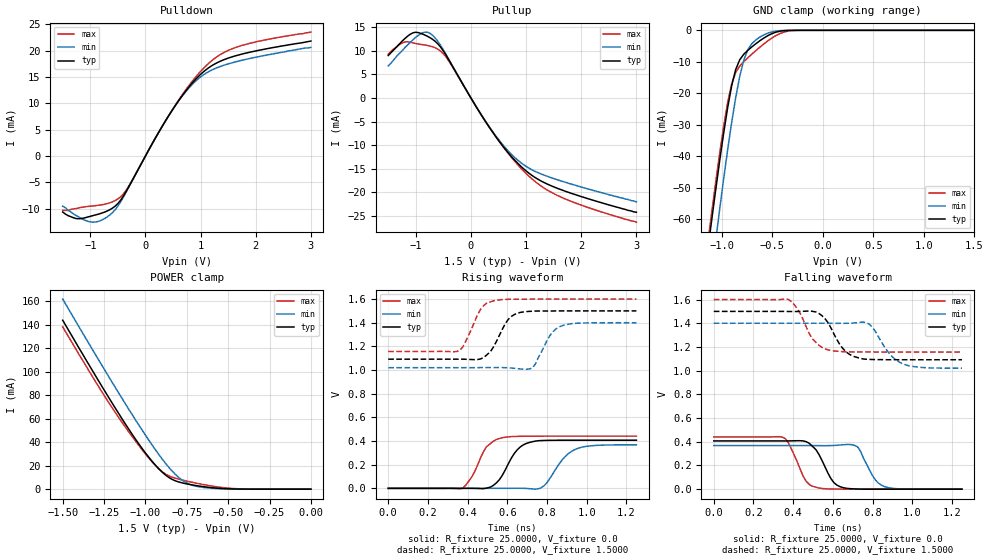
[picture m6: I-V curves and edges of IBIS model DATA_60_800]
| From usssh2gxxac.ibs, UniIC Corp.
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|   Model DATA_60_800
[Model]  DATA_60_800
Model_type I/O
Polarity   Non-Inverting
Enable   Active-High
Vinl =   0.60000000V
Vinh =   0.90000000V
Vmeas =   0.750000000V
Rref =   25.00000000
Vref =   0.75000000V
C_comp   1.6160pF   1.5990pF   1.6430pF
[Temperature Range]   25.0000   95.0000   0.0
[Voltage Range]   1.5000V   1.4000V   1.6000V
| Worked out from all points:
|   slope of the pulldown table from 0 to 0.225 V, typ, clamps not added: 53.4 ohm
|   slope of the pullup table from 0 to 0.225 V, typ, clamps not added: 52.6 ohm
|   GND clamp passes 1 mA (typ) near -0.50 V on its own axis
|   POWER clamp passes 1 mA (typ) near -0.58 V on its own axis
|   rising waveform, R_fixture 25.0000, V_fixture 0.0: 20-80 % time 86.5ps typ, 98.3ps min, 79.3ps max; typ from 0 V to 0.407 V
|   rising waveform, R_fixture 25.0000, V_fixture 1.5000: 20-80 % time 78.8ps typ, 76.2ps min, 73.4ps max; typ from 1.09 V to 1.5 V
|   falling waveform, R_fixture 25.0000, V_fixture 0.0: 20-80 % time 75.8ps typ, 70.4ps min, 70.8ps max; typ from 0.407 V to 0 V
|   falling waveform, R_fixture 25.0000, V_fixture 1.5000: 20-80 % time 88.4ps typ, 97.1ps min, 85.7ps max; typ from 1.5 V to 1.09 V
[Pulldown]
|Voltage   I(typ)   I(min)   I(max)
-1.5V     -10.6mA    -9.5mA     -10.3mA
-1.25V    -11.86mA   -11.3mA    -9.93mA
-1V       -11.42mA   -12.48mA   -9.5mA
-800mV    -10.84mA   -12.17mA   -9.25mA
-600mV    -9.882mA   -10.74mA   -8.682mA
-350mV    -6.704mA   -6.838mA   -6.505mA
200mV     3.763mA    3.796mA    3.76mA
550mV     9.696mA    9.684mA    9.781mA
850mV     13.86mA    13.59mA    14.19mA
1.15V     16.76mA    16.02mA    17.61mA
1.75V     19.33mA    18.16mA    20.97mA
3V        21.8mA     20.6mA     23.5mA
[Pullup]
|Voltage   I(typ)   I(min)   I(max)
-1.5V     9mA        6.8mA      9.3mA
-1.25V    12.03mA    10mA       11.63mA
-1.05V    13.82mA    12.36mA    11.68mA
-900mV    13.65mA    13.69mA    11.34mA
-750mV    12.84mA    13.77mA    11.04mA
-600mV    11.47mA    12.01mA    10.35mA
-450mV    9.041mA    9.198mA    8.665mA
300mV     -5.62mA    -5.548mA   -5.6mA
850mV     -13.84mA   -13.18mA   -14.16mA
1.2V      -17.1mA    -15.73mA   -18.03mA
1.55V     -19.04mA   -17.25mA   -20.54mA
3V        -24.2mA    -22mA      -26.3mA
[GND_clamp]
|Voltage   I(typ)   I(min)   I(max)
-1.5V     -169mA     -189.1mA   -163.8mA
-1.14V    -70.71mA   -88.3mA    -68.32mA
-1.1V     -60.74mA   -77.66mA   -58.33mA
-1.06V    -51.03mA   -67.22mA   -48.61mA
-1.02V    -41.65mA   -57.06mA   -39.27mA
-940mV    -24.55mA   -37.9mA    -22.88mA
-860mV    -12.39mA   -21.26mA   -13.32mA
-780mV    -7.577mA   -9.433mA   -9.942mA
-740mV    -6.329mA   -6.125mA   -8.71mA
-620mV    -3.273mA   -2.113mA   -5.305mA
-300mV    -11.81uA   -4.878uA   -91.71uA
1.5V      4.577nA    23.6nA     33.33nA
[POWER_clamp]
|Voltage   I(typ)   I(min)   I(max)
-1.5V     143.7mA    161.7mA    138.1mA
-1.22V    77.56mA    95.29mA    73.32mA
-1.12V    55.19mA    72.34mA    52.54mA
-1.02V    34.59mA    50.23mA    33.56mA
-960mV    23.77mA    37.63mA    23.28mA
-900mV    14.66mA    25.9mA     15mA
-840mV    8.415mA    15.63mA    10.28mA
-780mV    5.408mA    7.848mA    7.861mA
-700mV    3.206mA    2.693mA    5.332mA
-600mV    1.29mA     794.5uA    2.681mA
-420mV    69.47uA    44.47uA    238.7uA
0V        4.577nA    6.249nA    39.08nA
[Ramp]
| variable   typ   min   max
dV/dt_r  0.2442/86.5366p   0.2207/98.3857p   0.2647/78.9981p
dV/dt_f  0.2448/88.3671p   0.2280/97.6364p   0.2658/81.8205p
R_load = 25.0000
[Rising Waveform]
R_fixture= 25.0000
V_fixture= 0.0
V_fixture_min= 0.0
V_fixture_max= 0.0
|time   V(typ)   V(min)   V(max)
0s        0V         0V         0V
375ps     135.4uV    0V         1.139mV
515ps     10.65mV    -21.45uV   378.8mV
560ps     73.7mV     46.14uV    422mV
650ps     326.4mV    653.8uV    439.3mV
755ps     402.5mV    -3.935mV   441.1mV
800ps     405.5mV    49.9mV     441.2mV
890ps     406.9mV    267mV      441.2mV
950ps     407mV      335.2mV    441.2mV
1.25ns    407mV      367.8mV    441.2mV
[Rising Waveform]
R_fixture= 25.0000
V_fixture= 1.5000
V_fixture_min= 1.4000
V_fixture_max= 1.6000
|time   V(typ)   V(min)   V(max)
0s        1.092V     1.02V      1.157V
360ps     1.092V     1.02V      1.167V
465ps     1.094V     1.021V     1.513V
530ps     1.195V     1.021V     1.585V
605ps     1.429V     1.019V     1.598V
665ps     1.487V     1.009V     1.599V
725ps     1.497V     1.017V     1.6V
815ps     1.499V     1.293V     1.6V
860ps     1.5V       1.364V     1.6V
1.25ns    1.5V       1.4V       1.6V
[Falling Waveform]
R_fixture= 25.0000
V_fixture= 0.0
V_fixture_min= 0.0
V_fixture_max= 0.0
|time   V(typ)   V(min)   V(max)
0s        407mV      367.9mV    441.2mV
345ps     406.9mV    367.9mV    439.3mV
465ps     400.8mV    367.8mV    67.61mV
530ps     292.2mV    367.5mV    9.851mV
590ps     89.18mV    367.9mV    1.433mV
650ps     13.4mV     374.5mV    209.2uV
725ps     1.268mV    355.8mV    19.2uV
815ps     49.16uV    75.55mV    0V
860ps     11.86uV    21.72mV    0V
1.25ns    0V         1.289uV    0V
[Falling Waveform]
R_fixture= 25.0000
V_fixture= 1.5000
V_fixture_min= 1.4000
V_fixture_max= 1.6000
|time   V(typ)   V(min)   V(max)
0s        1.5V       1.4V       1.6V
375ps     1.499V     1.4V       1.602V
420ps     1.499V     1.4V       1.524V
515ps     1.495V     1.4V       1.238V
575ps     1.406V     1.399V     1.176V
665ps     1.161V     1.399V     1.16V
755ps     1.098V     1.409V     1.158V
800ps     1.094V     1.364V     1.158V
950ps     1.092V     1.059V     1.157V
1.25ns    1.092V     1.021V     1.157V
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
